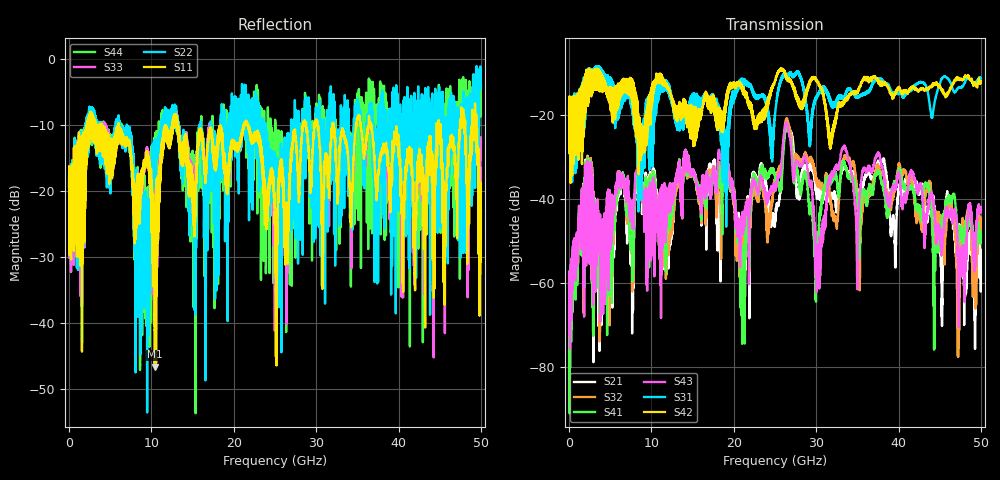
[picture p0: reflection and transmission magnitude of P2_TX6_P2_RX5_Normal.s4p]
!Keysight Technologies,N5225B,MY57041031,A.13.20.10
!Date: Friday, May 31, 2019 11:34:39
!Correction: S11(Full 4 Port(1,2,3,4))
!S12(Full 4 Port(1,2,3,4))
!S13(Full 4 Port(1,2,3,4))
!S14(Full 4 Port(1,2,3,4))
!S21(Full 4 Port(1,2,3,4))
!S22(Full 4 Port(1,2,3,4))
!S23(Full 4 Port(1,2,3,4))
!S24(Full 4 Port(1,2,3,4))
!S31(Full 4 Port(1,2,3,4))
!S32(Full 4 Port(1,2,3,4))
!S33(Full 4 Port(1,2,3,4))
!S34(Full 4 Port(1,2,3,4))
!S41(Full 4 Port(1,2,3,4))
!S42(Full 4 Port(1,2,3,4))
!S43(Full 4 Port(1,2,3,4))
!S44(Full 4 Port(1,2,3,4))
!S4P File: Measurements: <S11,S12,S13,S14>,
!<S21,S22,S23,S24>,
!<S31,S32,S33,S34>,
!<S41,S42,S43,S44>:
# Hz S  dB  R 50.0
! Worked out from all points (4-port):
!   5000 points, 10 MHz to 50 GHz, reference 50 ohm
!   strongest paths, dB at 10 MHz, 12.51 GHz, 25.01 GHz, 37.51 GHz, 50 GHz:
!     S42: -19.4, -16.9, -11.8, -11.4, -12.0
!     S31: -19.4, -16.8, -20.0, -11.6, -11.4
!     S43: -57.3, -41.2, -36.8, -28.9, -42.5
!     S41: -68.2, -43.5, -34.8, -33.5, -48.8
!     S32: -76.1, -45.2, -35.8, -32.1, -44.4
!     S21: -70.8, -46.0, -44.9, -30.9, -57.3
!   lowest |S11| = -46.6 dB at 10.41 GHz (marker M1), VSWR 1.01, Z = 50 - j0.464 ohm
!   |S11| at or under -10 dB: 13.21 GHz to 21.18 GHz (7.966 GHz wide, 46.3 % of centre); 21.74 GHz to 28.38 GHz (6.638 GHz wide, 26.5 % of centre); 36.67 GHz to 44.63 GHz (7.961 GHz wide, 19.6 % of centre)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
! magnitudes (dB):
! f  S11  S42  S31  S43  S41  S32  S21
! 10 MHz  -19.4  -19.4  -19.4  -57.3  -68.2  -76.1  -70.8
! 2.15 GHz  -14.6  -14.5  -16.8  -32.3  -31.4  -31.6  -31.1
! 10.41 GHz  -46.6  -12.9  -14.9  -51.4  -44.8  -40.5  -40.0
! 21.07 GHz  -10.9  -14.4  -11.8  -47.2  -68.8  -50.9  -55.3
! 26.52 GHz  -25.6  -11.7  -10.5  -22.5  -23.1  -21.3  -22.4
! 30.18 GHz  -10.2  -12.3  -15.1  -53.5  -49.5  -36.9  -39.0
! 50 GHz  -23.0  -12.0  -11.4  -42.5  -48.8  -44.4  -57.3
